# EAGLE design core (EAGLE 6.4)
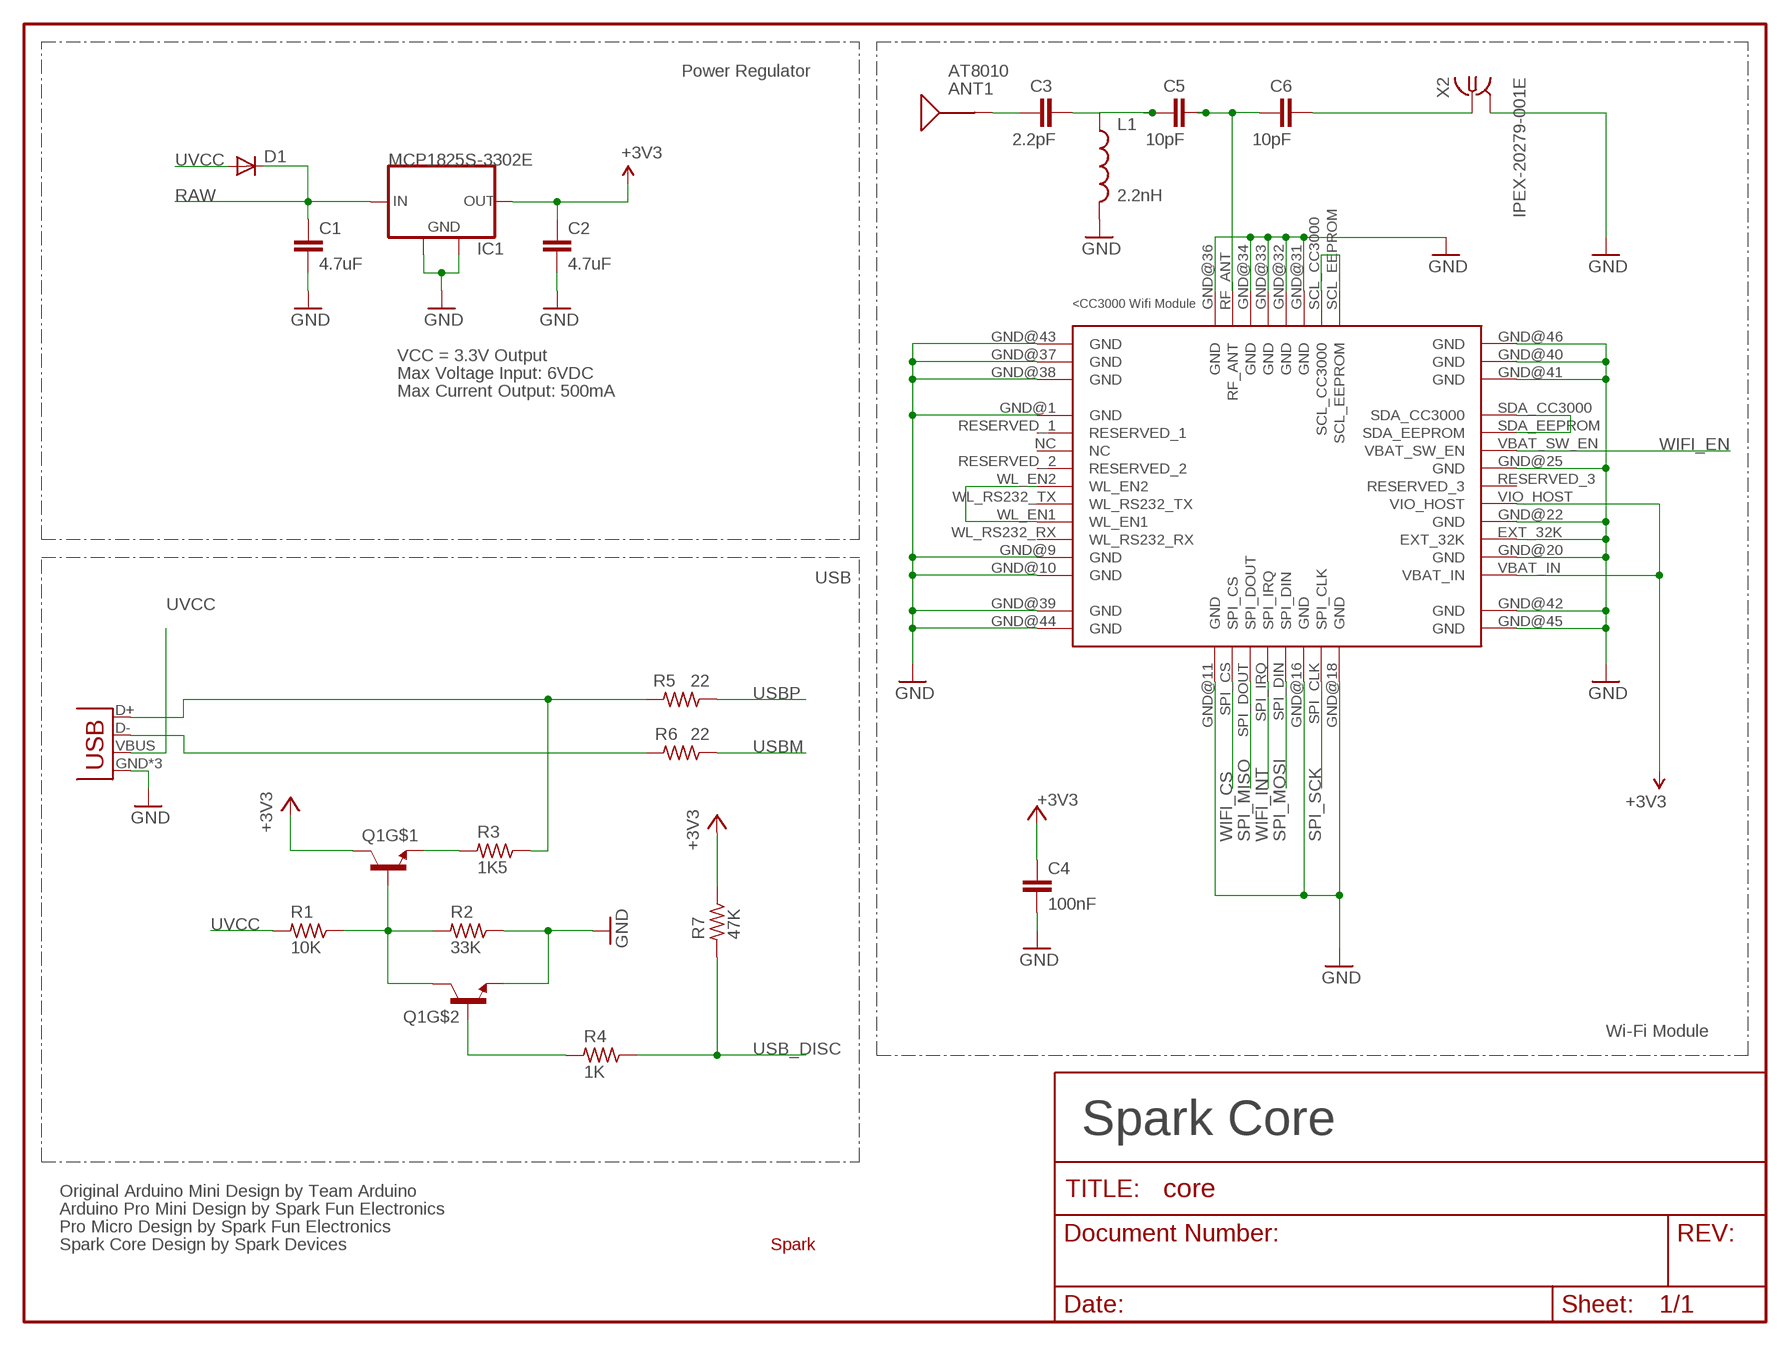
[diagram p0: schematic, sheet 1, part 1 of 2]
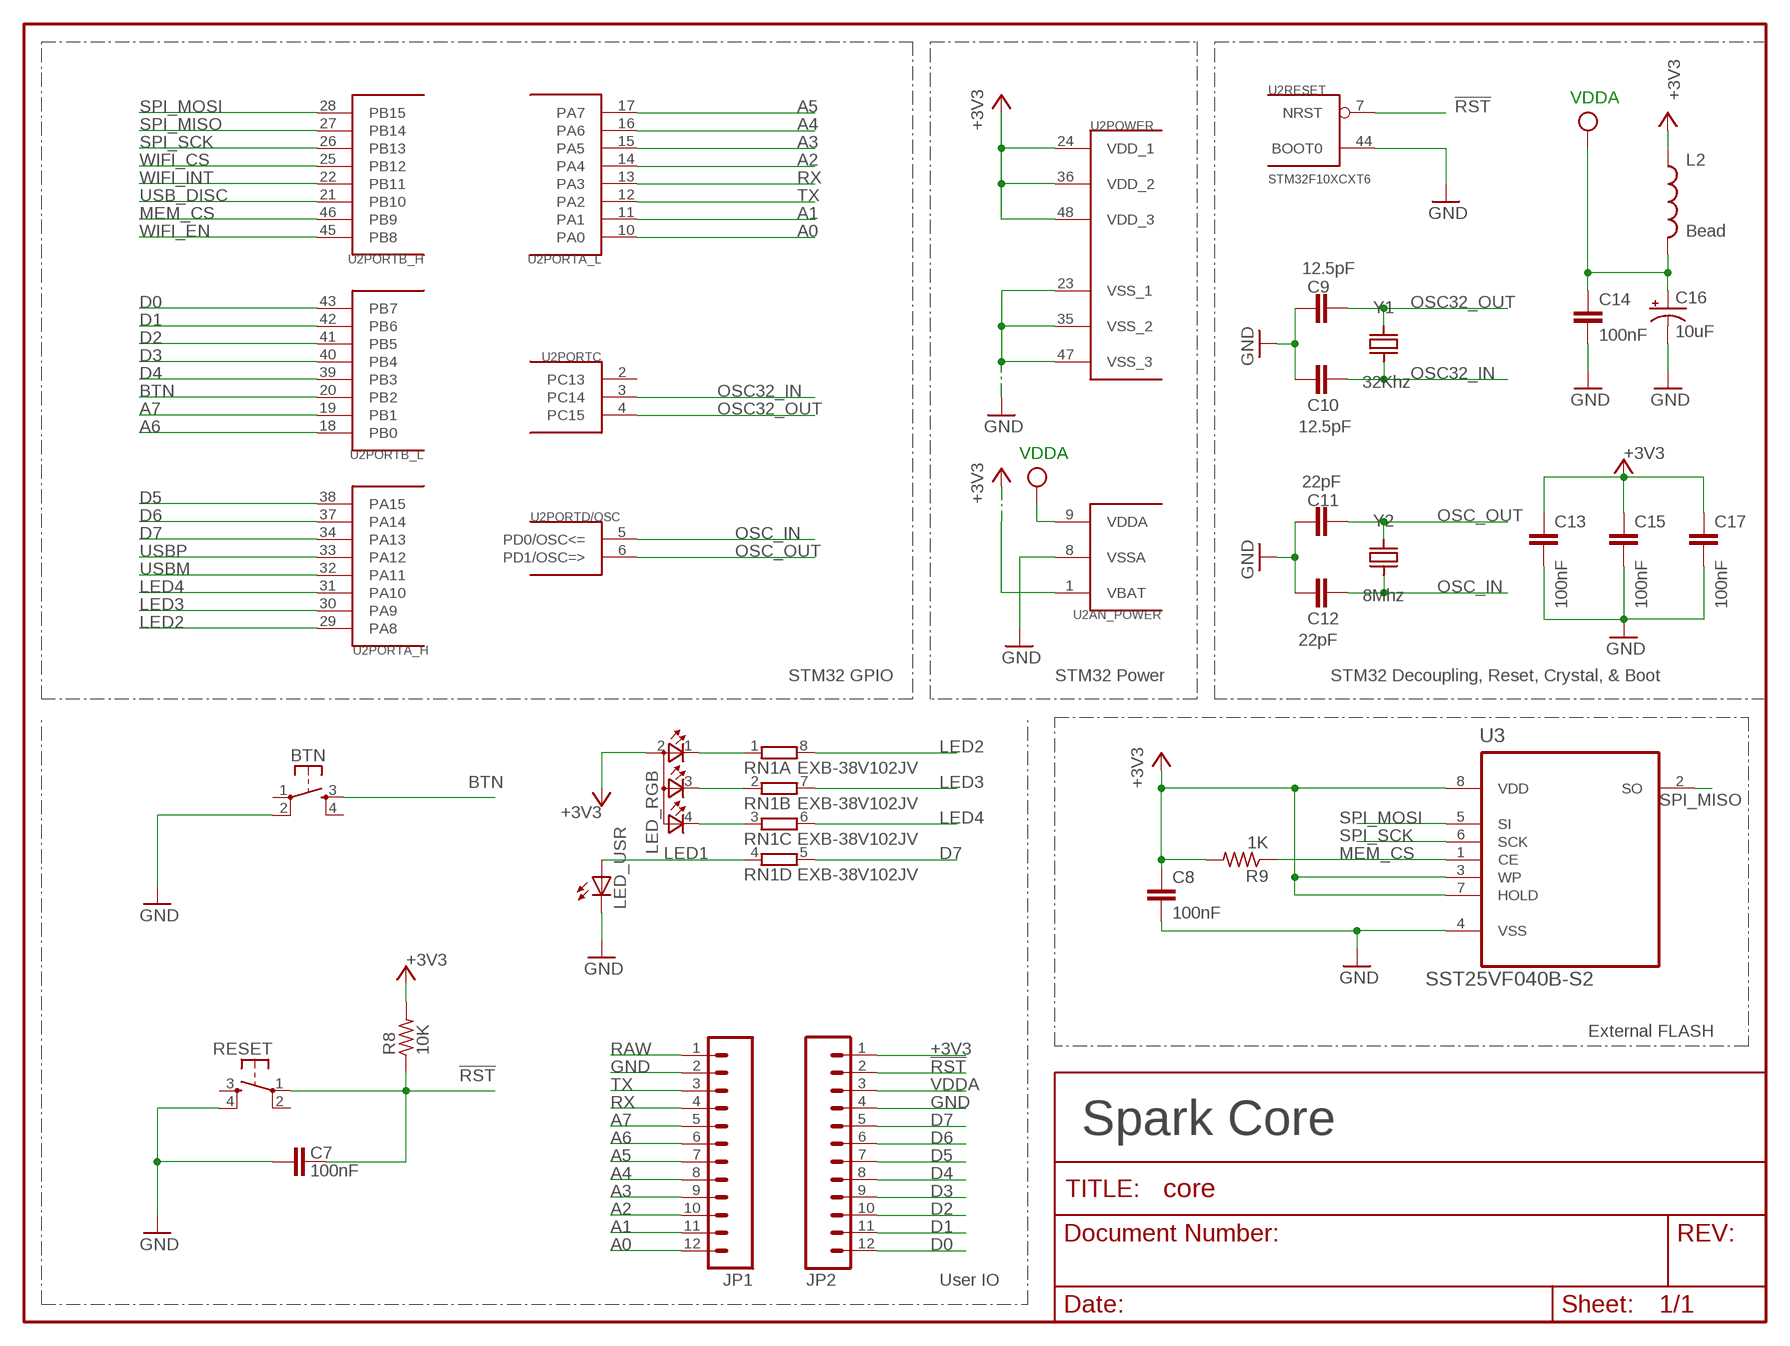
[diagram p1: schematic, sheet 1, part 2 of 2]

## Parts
ANT1  AT8010  [AT8010]
BTN  KMR211GLFS  TAC_SWITCHSMD  [TACTILE_SWITCH_SMD]
C1  4.7uF  C-EUC0603  [C0603]
C2  4.7uF  C-EUC0603  [C0603]
C3  2.2pF  C-EUC0603  [C0603]
C4  100nF  C-EUC0603  [C0603]
C5  10pF  C-EUC0603  [C0603]
C6  10pF  C-EUC0603  [C0603]
C7  100nF  C-EUC0603  [C0603]
C8  100nF  C-EUC0603  [C0603]
C9  12.5pF  C-EUC0603  [C0603]
C10  12.5pF  C-EUC0603  [C0603]
C11  22pF  C-EUC0603  [C0603]
C12  22pF  C-EUC0603  [C0603]
C13  100nF  C-EUC0603  [C0603]
C14  100nF  C-EUC0603  [C0603]
C15  100nF  C-EUC0603  [C0603]
C16  10uF  TANT-CAP1206  [EIA3216]
C17  100nF  C-EUC0603  [C0603]
D1  DIODESOD  [SOD-323]
IC1  MCP1825S-3302E  MCP1825S-SOT223  [SOT223]
JP1  M12PTH  [1X12]
JP2  M12PTH  [1X12]
L1  2.2nH  INDUCTOR0603  [0603]
L2  Bead  INDUCTOR0603  [0603]
LED_RGB  TOPLED-3PLCC  [P-LCC-4-3]
LED_USR  LED0603  [LED-0603]
Q1  MMDT3904  [SOT363]
R1  10K  R-US_R0603  [R0603]
R2  33K  R-US_R0603  [R0603]
R3  1K5  R-US_R0603  [R0603]
R4  1K  R-US_R0603  [R0603]
R5  22  R-US_R0603  [R0603]
R6  22  R-US_R0603  [R0603]
R7  47K  R-US_R0603  [R0603]
R8  10K  R-US_R0603  [R0603]
R9  1K  R-US_R0603  [R0603]
RESET  KMR211GLFS  TAC_SWITCHSMD  [TACTILE_SWITCH_SMD]
RN1  EXB-38V102JV  4R-NEXB38V  [EXB38V]
U1  CC3000  [CC3000]
U2  STM32F10XCXT6  [TQFP48]
U3  SST25VF040B-S2  [SOIC127P790X216-8N]
U$1  SPARK_LOGO2  [SPARK_LOGO2]
X1  USB-MICROB  USBUSB-MICROB-ALIGN  [USB-MICROB-ALIGN]
X2  IPEX-20279-001E  [IPEX-20279-001E]
Y1  32Khz  Q_FC135  [FC135]
Y2  8Mhz  Q_3.2X2.5  [OSC3.2X.2.5]

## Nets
!RST: C7.2 JP2.2 R8.1 RESET.1 U2.7(RESET:NRST)
+3V3: C2.1 C4.1 C8.1 C13.1 C15.1 C17.1 IC1.3(OUT) JP2.1 L2.1 LED_RGB.2(A2) Q1.3(C) R7.1 R8.2 R9.2 U1.VBAT_IN U1.VIO_HOST U2.1(AN_POWER:VBAT) U2.24(POWER:VDD_1) U2.36(POWER:VDD_2) U2.48(POWER:VDD_3) U3.3(WP) U3.7(HOLD) U3.8(VDD)
A0: JP1.12 U2.10(PORTA_L:PA0)
A1: JP1.11 U2.11(PORTA_L:PA1)
A2: JP1.10 U2.14(PORTA_L:PA4)
A3: JP1.9 U2.15(PORTA_L:PA5)
A4: JP1.8 U2.16(PORTA_L:PA6)
A5: JP1.7 U2.17(PORTA_L:PA7)
A6: JP1.6 U2.18(PORTB_L:PB0)
A7: JP1.5 U2.19(PORTB_L:PB1)
BTN: BTN.3 U2.20(PORTB_L:PB2)
D0: JP2.12 U2.43(PORTB_L:PB7)
D1: JP2.11 U2.42(PORTB_L:PB6)
D2: JP2.10 U2.41(PORTB_L:PB5)
D3: JP2.9 U2.40(PORTB_L:PB4)
D4: JP2.8 U2.39(PORTB_L:PB3)
D5: JP2.7 U2.38(PORTA_H:PA15)
D6: JP2.6 U2.37(PORTA_H:PA14)
D7: JP2.5 RN1.5 U2.34(PORTA_H:PA13)
GND [vcc]: BTN.2 C1.2 C2.2 C4.2 C7.1 C8.2 C9.2 C10.2 C11.2 C12.2 C13.2 C14.2 C15.2 C16.C(-) C17.2 IC1.2(GND) IC1.4(GND) JP1.2 JP2.4 L1.2 LED_USR.C Q1.1(E) R2.1 RESET.4 U1.EXT_32K U1.GND@1(GND) U1.GND@9(GND) U1.GND@10(GND) U1.GND@11(GND) U1.GND@16(GND) U1.GND@18(GND) U1.GND@20(GND) U1.GND@22(GND) U1.GND@25(GND) U1.GND@31(GND) U1.GND@32(GND) U1.GND@33(GND) U1.GND@34(GND) U1.GND@36(GND) U1.GND@37(GND) U1.GND@38(GND) U1.GND@39(GND) U1.GND@40(GND) U1.GND@41(GND) U1.GND@42(GND) U1.GND@43(GND) U1.GND@44(GND) U1.GND@45(GND) U1.GND@46(GND) U2.8(AN_POWER:VSSA) U2.23(POWER:VSS_1) U2.35(POWER:VSS_2) U2.44(RESET:BOOT0) U2.47(POWER:VSS_3) U3.4(VSS) X1.GND X1.MT1(GND) X1.MT2(GND) X2.2@1(GND) X2.2@2(GND)
LED1: LED_USR.A RN1.4
LED2: RN1.8 U2.29(PORTA_H:PA8)
LED3: RN1.7 U2.30(PORTA_H:PA9)
LED4: RN1.6 U2.31(PORTA_H:PA10)
MEM_CS: R9.1 U2.46(PORTB_H:PB9) U3.1(CE)
N$1: R3.1 R5.2 X1.D+
N$2 [RF]: C6.2 X2.1
N$3 [RF]: ANT1.SIG(SIGNAL) C3.1
N$4 [RF]: C5.2 C6.1 U1.RF_ANT
N$5 [RF]: C3.2 C5.1 L1.1
N$6: R6.2 X1.D-
N$7: U1.SCL_CC3000 U1.SCL_EEPROM
N$8: Q1.2(B) R4.2
N$9: U1.WL_EN1 U1.WL_EN2
N$10: LED_RGB.1(CRED) RN1.1
N$12: LED_RGB.3(CBLUE) RN1.2
N$13: Q1.5(B) Q1.6(C) R1.1 R2.2
N$14: LED_RGB.4(CGREEN) RN1.3
N$15: U1.SDA_CC3000 U1.SDA_EEPROM
N$16: Q1.4(E) R3.2
OSC32_IN: C10.1 U2.3(PORTC:PC14) Y1.X1
OSC32_OUT: C9.1 U2.4(PORTC:PC15) Y1.X2
OSC_IN: C12.1 U2.5(PORTD/OSC:PD0/OSC<=) Y2.P$1
OSC_OUT: C11.1 U2.6(PORTD/OSC:PD1/OSC=>) Y2.P$3
RAW [vcc]: C1.1 D1.1(C) IC1.1(IN) JP1.1
RX: JP1.4 U2.13(PORTA_L:PA3)
SPI_MISO: U1.SPI_DOUT U2.27(PORTB_H:PB14) U3.2(SO)
SPI_MOSI: U1.SPI_DIN U2.28(PORTB_H:PB15) U3.5(SI)
SPI_SCK: U1.SPI_CLK U2.26(PORTB_H:PB13) U3.6(SCK)
TX: JP1.3 U2.12(PORTA_L:PA2)
USB_DISC: R4.1 R7.2 U2.21(PORTB_H:PB10)
USBM: R6.1 U2.32(PORTA_H:PA11)
USBP: R5.1 U2.33(PORTA_H:PA12)
UVCC: D1.2(A) R1.2 X1.VBUS
VDDA: C14.1 C16.A(+) JP2.3 L2.2 U2.9(AN_POWER:VDDA) ; supply symbol labelled VCC
WIFI_CS: U1.SPI_CS U2.25(PORTB_H:PB12)
WIFI_EN: U1.VBAT_SW_EN U2.45(PORTB_H:PB8)
WIFI_INT: U1.SPI_IRQ U2.22(PORTB_H:PB11)
Unconnected: BTN.1 BTN.4 RESET.2 RESET.3 U1.NC U1.RESERVED_1 U1.RESERVED_2 U1.RESERVED_3 U1.WL_RS232_RX U1.WL_RS232_TX U2.2(PORTC:PC13)

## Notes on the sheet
- Power Regulator
- VDDA
- VCC = 3.3V Output
- Max Voltage Input: 6VDC
- Max Current Output: 500mA
- VDDA
- USB
- STM32 GPIO | STM32 Power | STM32 Decoupling, Reset, Crystal, & Boot
- Wi-Fi Module | External FLASH
- Spark Core | Spark Core
- Original Arduino Mini Design by Team Arduino
- Arduino Pro Mini Design by Spark Fun Electronics
- Pro Micro Design by Spark Fun Electronics
- Spark Core Design by Spark Devices
- User IO

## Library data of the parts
ANT1 = Spark:AT8010: AT8010 Series Multilayer Chip Antenna
BTN RESET = Spark:TAC_SWITCH: SMD Tactiile Switch
C1-C15 C17 = rcl:C-EU: CAPACITOR, European symbol
C16 = Spark:TANT-CAP: Tantalum SMT
D1 = SparkFun:DIODE: Diode
IC1 = Spark:MCP1825S: 500 mA, Low Voltage, Low Quiescent Current LDO Regulator
JP1 JP2 = SparkFun:M12: Header 12 Standard 12-pin 0.1" header. Use with straight break away headers (SKU : PRT-00116), right angle break away headers (PRT-00553), swiss pins (PRT-00743), machine pins (PRT-00117), and female headers (PRT-00115).
L1 L2 = SparkFun-Passives:INDUCTOR: Inductors
LED_RGB = Spark:TOPLED-3: Cree CLVBA-FKA
LED_USR = SparkFun:LED: LEDs
Q1 = SparkFun-DiscreteSemi:MMDT3904: Dual NPN transistor
R1-R9 = rcl:R-US_: RESISTOR, American symbol
RN1 = resistor-dil:4R-N: Array Chip Resistor Source: RS Component / Phycomp; OC_FARNELL: unknown; OC_NEWARK: unknown
U1 = CC3000:CC3000
U2 = stm32:STM32F10XCXT6: ST STM32F101/103 48pin LQFP
U3 = Spark:SST25VF040B: 4 Mbit SPI Serial Flash
U$1 = Spark:SPARK_LOGO2
X1 = Spark:USB: USB Connectors USB-B-PTH is fully proven SKU : PRT-00139/CONN-08278 USB-miniB is fully proven SKU : PRT-00587 USB-A-PCB is untested. USB-A-H is throughly reviewed, but untested. Spark Fun Electronics SKU : PRT-00437 USB-B-SMT is throughly reviewed, but untested. Needs silkscreen touching up.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
X2 = Spark:IPEX-20279-001E: Ultra Miniature Coaxial SMT RF Receptacle
Y1 Y2 = Spark:Q

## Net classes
2 RF: width 0.635 mm, clearance 0.762 mm

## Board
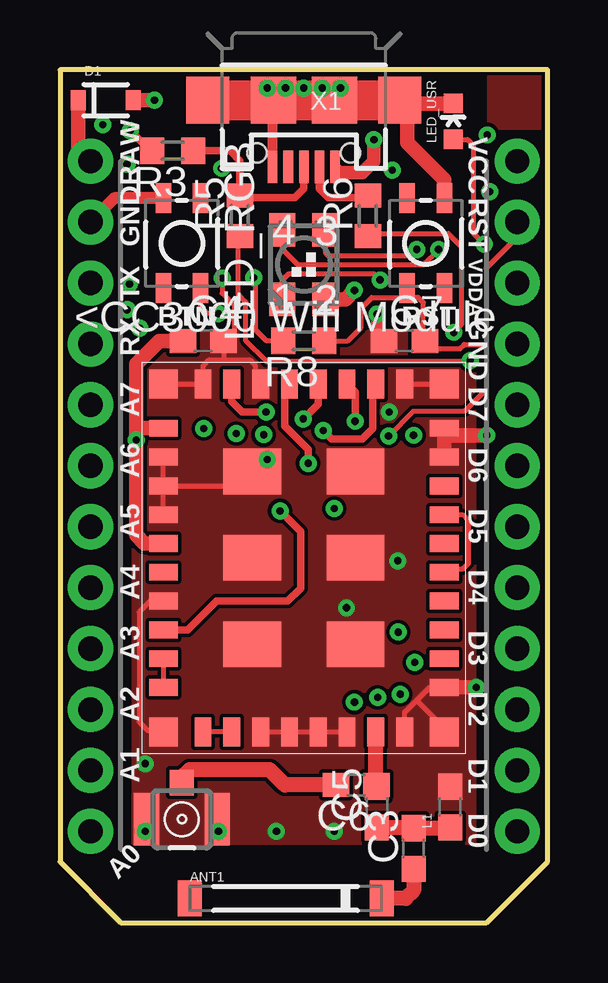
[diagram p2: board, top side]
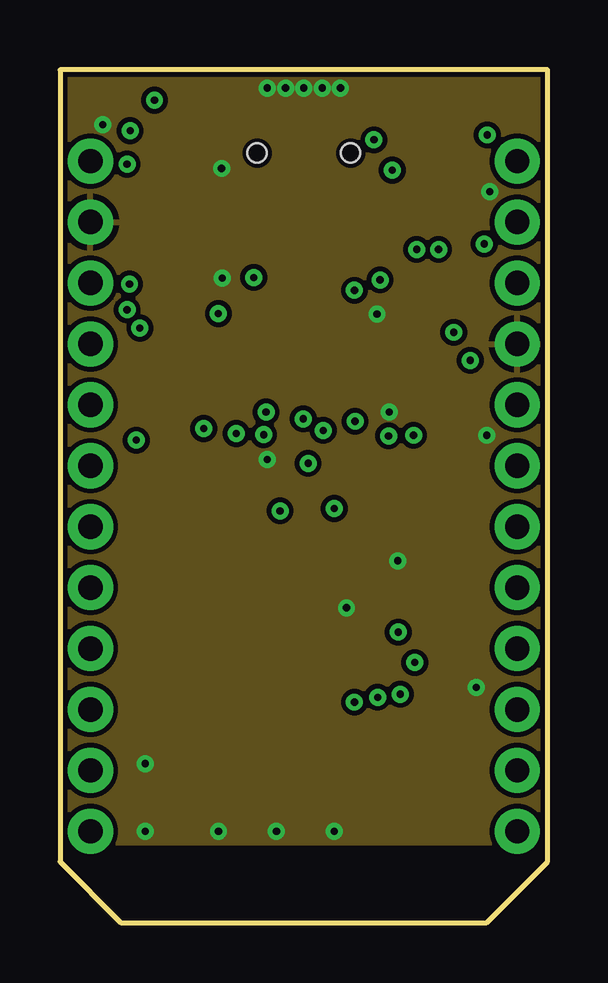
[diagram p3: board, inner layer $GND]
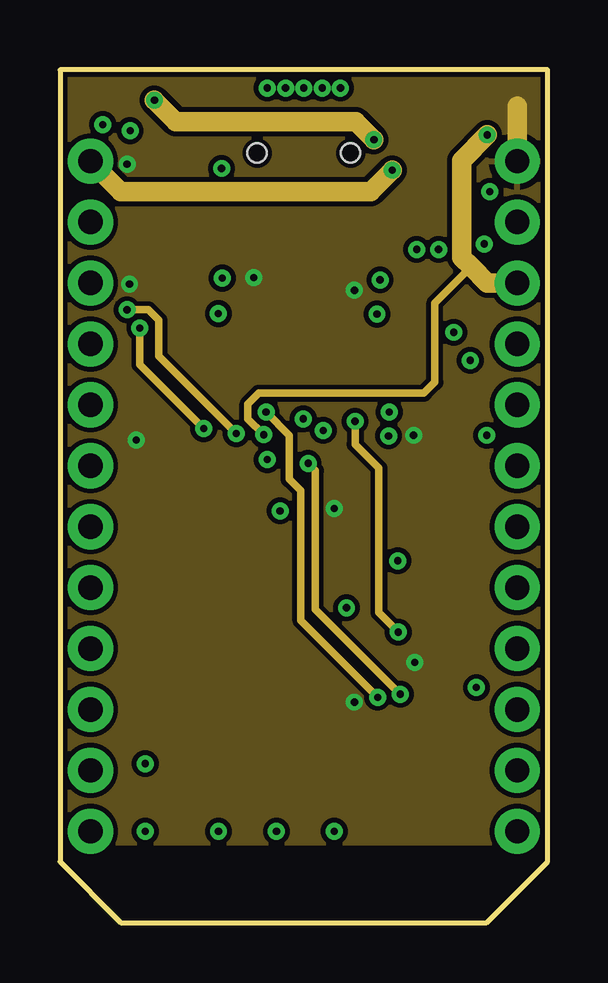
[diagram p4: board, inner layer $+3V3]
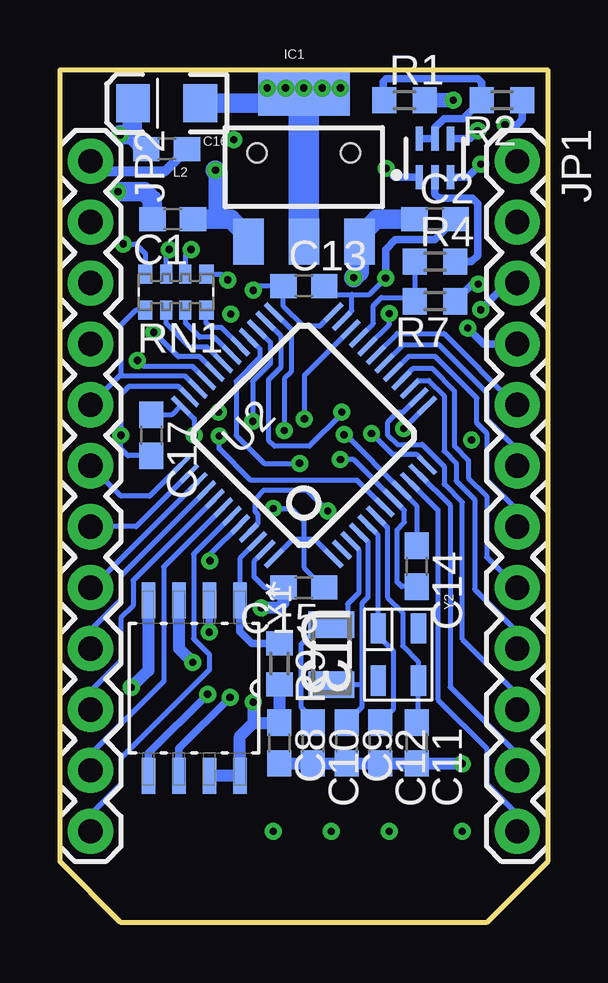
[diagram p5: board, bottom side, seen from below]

Size 20.32 x 35.56 mm. Coordinates in mm from the lower left corner, seen from the top.
Outline: 0,35.56 0,2.54 2.54,0 17.78,0 20.32,2.54 20.32,35.56 0,35.56
Copper layers (1+2*15+16): Top 0.035mm / dielectric 1.5mm / $GND 0.035mm / dielectric 0.15mm / $+3V3 0.035mm / dielectric 0.2mm / Bottom 0.035mm
Design rules "spark": minimum track width 6mil, minimum drill 0.3mm, track to track 6mil, track to pad 6mil, pad to pad 6mil, via to via 6mil, smd to smd 6mil, copper to edge 6mil, drill to drill 6mil, minimum pad ring 12mil, minimum via ring 8mil, stop-mask expansion 4mil, vias tented up to drill 20mil, thermal gap 10mil

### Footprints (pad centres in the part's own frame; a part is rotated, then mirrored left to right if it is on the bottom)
AT8010 = smd 1 x 1.5: NC -4,0; SIG 4,0
TACTILE_SWITCH_SMD = smd 1.25 x 0.65: 1 -1.875,0.775; 2 1.875,0.775; 3 -1.875,-0.775; 4 1.875,-0.775
C0603 = smd 1.1 x 1: 1 -0.85,0; 2 0.85,0
EIA3216 = smd 1.4 x 1.6: A 1.4,0; C -1.4,0
SOD-323 = smd 0.63 x 0.83: 1 -1.15,0; 2 1.15,0
SOT223 = smd 1.27 x 1.905: 1 -2.311,-3.099; 2 0,-3.099; 3 2.311,-3.099 | smd 3.81 x 1.905: 4 0,3.099
1X12 = drill 1.016 pad 1.88: 1 0,0; 2 2.54,0; 3 5.08,0; 4 7.62,0; 5 10.16,0; 6 12.7,0; 7 15.24,0; 8 17.78,0; 9 20.32,0; 10 22.86,0; 11 25.4,0; 12 27.94,0
0603 = smd 1.1 x 1: 1 -0.85,0; 2 0.85,0
P-LCC-4-3 = smd 1.1 x 1.4: 1 -0.9,-1.45; 2 0.9,-1.45; 3 0.9,1.45; 4 -0.9,1.45
LED-0603 = smd 0.8 x 0.8: A 0,-0.75; C 0,0.75
SOT363 = smd 0.3 x 0.99: 1 -0.65,-0.8; 2 0,-0.8; 3 0.65,-0.8; 4 0.65,0.81; 5 0,0.81; 6 -0.65,0.81
R0603 = smd 1 x 1.1: 1 -0.85,0; 2 0.85,0
EXB38V = smd 0.6 x 0.8: 1 -1.275,-0.75; 4 1.275,-0.75; 5 1.275,0.75; 8 -1.275,0.75 | smd 0.5 x 0.8: 2 -0.4,-0.75; 3 0.4,-0.75; 6 0.4,0.75; 7 -0.4,0.75
CC3000 = smd 1.2 x 0.7: EXT_32K 5.85,-2.97; GND@1 -5.85,5.43; GND@9 -5.85,-4.17; GND@10 -5.85,-5.37; GND@20 5.85,-4.17; GND@22 5.85,-1.77; GND@25 5.85,1.83; NC -5.85,3.03; RESERVED_1 -5.85,4.23; RESERVED_2 -5.85,1.83; RESERVED_3 5.85,0.63; SDA_CC3000 5.85,5.43; SDA_EEPROM 5.85,4.23; VBAT_IN 5.85,-5.37; VBAT_SW_EN 5.85,3.03; VIO_HOST 5.85,-0.57; WL_EN1 -5.85,-1.77; WL_EN2 -5.85,0.63; WL_RS232_RX -5.85,-2.97; WL_RS232_TX -5.85,-0.57 | smd 0.7 x 1.2: GND@11 -4.2,-7.22; GND@16 1.8,-7.22; GND@18 4.2,-7.22; GND@31 1.8,7.28; GND@32 0.6,7.28; GND@33 -0.6,7.28; GND@34 -1.8,7.28; GND@36 -4.2,7.28; RF_ANT -3,7.28; SCL_CC3000 3,7.28; SCL_EEPROM 4.2,7.28; SPI_CLK 3,-7.22; SPI_CS -3,-7.22; SPI_DIN 0.6,-7.22; SPI_DOUT -1.8,-7.22; SPI_IRQ -0.6,-7.22 | smd 2.4 x 1.9: GND@37 -2.15,3.63; GND@38 -2.15,0.03; GND@39 -2.15,-3.57; GND@40 2.15,3.63; GND@41 2.15,0.03; GND@42 2.15,-3.57 | smd 1.2 x 1.2: GND@43 -5.85,7.28; GND@44 -5.85,-7.22; GND@45 5.85,-7.22; GND@46 5.85,7.28
TQFP48 = smd 0.2 x 1: 1 -2.75,-4.5; 2 -2.25,-4.5; 3 -1.75,-4.5; 4 -1.25,-4.5; 5 -0.75,-4.5; 6 -0.25,-4.5; 7 0.25,-4.5; 8 0.75,-4.5; 9 1.25,-4.5; 10 1.75,-4.5; 11 2.25,-4.5; 12 2.75,-4.5; 25 2.75,4.5; 26 2.25,4.5; 27 1.75,4.5; 28 1.25,4.5; 29 0.75,4.5; 30 0.25,4.5; 31 -0.25,4.5; 32 -0.75,4.5; 33 -1.25,4.5; 34 -1.75,4.5; 35 -2.25,4.5; 36 -2.75,4.5 | smd 1 x 0.2: 13 4.5,-2.75; 14 4.5,-2.25; 15 4.5,-1.75; 16 4.5,-1.25; 17 4.5,-0.75; 18 4.5,-0.25; 19 4.5,0.25; 20 4.5,0.75; 21 4.5,1.25; 22 4.5,1.75; 23 4.5,2.25; 24 4.5,2.75; 37 -4.5,2.75; 38 -4.5,2.25; 39 -4.5,1.75; 40 -4.5,1.25; 41 -4.5,0.75; 42 -4.5,0.25; 43 -4.5,-0.25; 44 -4.5,-0.75; 45 -4.5,-1.25; 46 -4.5,-1.75; 47 -4.5,-2.25; 48 -4.5,-2.75
SOIC127P790X216-8N = smd 1.499 x 0.559: 1 -3.658,1.905; 2 -3.658,0.635; 3 -3.658,-0.635; 4 -3.658,-1.905; 5 3.658,-1.905; 6 3.658,-0.635; 7 3.658,0.635; 8 3.658,1.905
USB-MICROB-ALIGN = smd 0.4 x 1.35: D+ 0,2.775; D- -0.65,2.775; GND 1.3,2.775; ID 0.65,2.775; VBUS -1.3,2.775 | smd 1.8 x 1.95: MT1 -4,0; MT2 4,0 | smd 1.9 x 1.95: P$1 -1.27,0; P$2 1.27,0 | hole 0.8: -1.95,2.2; 1.95,2.2
IPEX-20279-001E = smd 1 x 1.05: 1 0,1.528 | smd 1.05 x 2.2: 2@1 -1.475,0; 2@2 1.475,0
FC135 = smd 1.1 x 1.9: X1 -1.25,0; X2 1.25,0
OSC3.2X.2.5 = smd 1.27 x 0.635: P$1 -1.092,-0.838; P$2 1.092,-0.838; P$3 1.092,0.838; P$4 -1.092,0.838

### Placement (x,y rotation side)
ANT1  9.4,1.02 0 top
BTN  5.08,28.32 90 top
C1  15.62,29.34 180 bottom
C2  4.7,29.34 0 bottom
C3  14.73,3.1 90 top
C4  5.97,24.26 0 top
C5  13.21,4.83 90 top
C6  12.34,5.74 180 top
C7  14.35,24.26 0 top
C8  11.18,7.49 270 bottom
C9  8.38,7.49 270 bottom
C10  9.78,7.49 270 bottom
C11  5.46,7.49 270 bottom
C12  6.99,7.49 270 bottom
C13  10.16,26.54 0 bottom
C14  5.46,14.86 270 bottom
C15  10.16,13.97 180 bottom
C16  15.88,34.16 180 bottom
C17  16.51,20.32 270 bottom
D1  1.91,34.29 0 top
IC1  10.16,31.5 0 bottom
JP1  1.27,31.75 270 bottom
JP2  19.05,31.75 270 bottom
L1  16.26,4.83 90 top
L2  15.88,32.26 180 bottom
LED_RGB  10.16,27.43 0 top
LED_USR  16.38,33.4 0 top
Q1  4.7,31.88 0 bottom
R1  5.97,34.29 0 bottom
R2  1.91,34.29 180 bottom
R3  4.7,32.18 180 top
R4  4.7,27.56 0 bottom
R5  7.49,29.46 90 top
R6  12.83,29.46 90 top
R7  4.7,25.91 180 bottom
R8  10.16,24.26 180 top
R9  11.18,10.8 270 bottom
RESET  15.24,28.32 90 top
RN1  15.49,26.29 180 bottom
U1  10.16,15.24 180 top
U2  10.16,20.32 45 bottom
U3  14.73,9.78 270 bottom
U$1  17.78,33.02 0 top
X1  10.16,34.29 180 top
X2  5.08,4.32 0 top
Y1  9.02,11.18 270 bottom
Y2  6.22,11.18 270 bottom

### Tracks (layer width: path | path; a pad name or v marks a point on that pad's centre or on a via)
!RST  (via drill 0.3)
  Top 0.203: 17.75,24.08 17.75,27.28 19.05,28.57 JP2.2 | 17.75,24.08 17.75,22.22 16.84,21.31 14.71,21.31 v13.69,20.29 | 17.75,24.08 17.73,24.11 16.84,24.11 16.66,23.93 15.53,23.93 C7.2 15.14,24.32 15.14,25.86 14.94,26.06 14.46,26.06 | R8.1 11.99,24.26 12.55,24.82 12.55,25.63 12.98,26.06 14.46,26.06 | 14.46,26.06 RESET.1
  Bottom 0.203: U2.7 7.93,18.44 12.37,18.44 13.69,19.76 v13.69,20.29
+3V3  (via drill 0.3)
  Top 0.203: R8.2 8.61,24.26 8.15,24.71 8.15,26.82 v8.08,26.9
  Top 0.61: U1.VIO_HOST 3.52,15.81 3.17,16.15 v3.17,20.12 3.17,20.62 | 3.17,20.62 3.17,23.29 4.14,24.26 C4.1 | U1.VBAT_IN 4.29,20.62 3.17,20.62 | LED_RGB.2 11.88,25.98 v12.27,26.36
  $+3V3 0.813: JP2.1 19.05,34.04
  Bottom 0.203: U2.1 9.71,15.98 10.16,15.98 | 10.16,15.98 10.62,15.98 U2.48 | v11.43,17.27 10.69,17.27 10.16,16.74 10.16,15.98 | 9.32,13.97 C15.1 10.16,14.82 10.16,15.98 | v12.27,26.36 12.09,26.54 C13.1 11.01,25.69 10.19,24.87 9.5,24.87 U2.24 | C17.1 15.67,21.17 U2.36 14.73,21 v14.73,20.32
  Bottom 0.305: R7.1 3.14,26.62 v2.9,26.62 | Q1.3 3.34,31.08 v2.79,31.62
  Bottom 0.406: L2.1 15.96,31.32 18.62,31.32 JP2.1
  Bottom 0.508: 12.27,8.33 12.83,7.77 U3.8 U3.7 | 12.27,8.33 C8.1 R9.2 | v12.27,9.2 12.27,8.33 | U3.3 15.37,11.43 v14.78,10.85
  Bottom 0.813: C2.1 7.11,29.34 7.85,28.6 IC1.3 7.85,27.13 v8.08,26.9
  pour $+3V3 (isolate 0.203): 0,35.56 20.32,35.56 20.32,3.3 0,3.3
A0
  Bottom 0.203: U2.10 4.57,17.21 4.57,9.3 2.54,7.26 2.54,5.79 1.27,4.52 JP1.12
A1
  Bottom 0.203: U2.11 4.06,17.41 4.06,9.83 1.27,7.04 JP1.11
A2
  Bottom 0.203: U2.14 6.04,21.26 6.27,21.26 6.66,20.88 6.66,20.32 6.27,19.94 5.23,19.94 4.32,19.02 4.32,18.29 3.56,17.53 3.56,11.81 1.27,9.53 JP1.10
A3
  Bottom 0.203: U2.15 5.4,22.61 4.95,22.61 4.32,21.97 4.32,19.66 3.81,19.15 3.81,18.41 3.05,17.65 3.05,13.89 1.27,12.12 JP1.9
A4
  Bottom 0.203: U2.16 5.6,23.11 4.83,23.11 3.89,22.17 3.89,19.86 3.3,19.28 3.3,18.54 2.54,17.78 2.54,15.24 JP1.8
A5
  Bottom 0.203: U2.17 5.8,23.62 4.7,23.62 2.95,21.87 2.95,20.83 2.54,20.42 2.54,18.47 1.27,17.2 JP1.7
A6
  Bottom 0.203: U2.18 6.02,24.11 4.55,24.11 2.54,22.1 2.54,21.01 1.27,19.74 JP1.6
A7
  Bottom 0.203: U2.19 6.27,24.56 4.32,24.56 1.35,21.59 JP1.5
BTN  (via drill 0.3)
  Top 0.203: 5.84,26.43 BTN.3 5.87,26.43 5.87,25.65 6.13,25.39 v6.6,25.39
  Bottom 0.203: U2.20 6.6,24.94 v6.6,25.39
D0
  Bottom 0.203: U2.43 14.76,15.37 14.76,11.84 14.1,11.18 14.1,10.54 17.78,6.86 17.78,5.77 19.05,4.5 JP2.12
D1
  Bottom 0.203: U2.42 16,14.83 16,10.06 19.05,7.01 JP2.11
D2
  Bottom 0.203: JP2.10 19.05,9.65 17.78,10.92 17.78,12.7 17.27,13.21 17.27,14.27 U2.41
D3
  Bottom 0.203: JP2.9 19.05,12.19 17.78,13.46 17.78,14.48 17.77,14.48 U2.40
D4
  Bottom 0.203: U2.39 18.98,13.97 JP2.8
D5
  Bottom 0.203: JP2.7 17.15,16.51 U2.38
D6
  Bottom 0.203: U2.37 16.59,17.78 17.78,17.78 JP2.6
D7
  Bottom 0.203: U2.34 15.1,22.78 17.86,22.78 | 17.86,22.78 JP2.5 | RN1.5 17.16,25.54 17.78,24.92 17.78,22.86 17.86,22.78
GND  (via drill 0.3)
  Top 0.203: U1.GND@43 16.01,8.12 14.86,9.27 | U1.GND@36 14.36,8.77 14.86,9.27 | U1.GND@1 15.4,9.81 14.86,9.27 | v8.64,19.3 8.14,18.81 U1.GND@42 7.41,18.21 U1.EXT_32K | U1.GND@34 U1.GND@33 U1.GND@32 U1.GND@31 8.36,8.4 | U1.GND@22 U1.EXT_32K | U1.GND@45 U1.GND@18 | U1.GND@38 12.41,15.11 | U1.GND@25 4.49,13.59 3.94,13.59 3.3,12.95 3.3,8.38 3.68,8 4.27,8 U1.GND@46 | U1.GND@11 U1.GND@44 | U1.EXT_32K U1.GND@20 | U1.GND@18 | 8.26,21.97 8.26,22.36 U1.GND@16 8.13,22.69 8.13,23.24 7.9,23.47 6.83,23.47 | 6.22,34.23 X1.MT2 | U1.GND@18 5.96,23.21 6.22,23.47 6.83,23.47 | 6.83,23.47 6.82,23.48 C4.2 7.26,24.7 7.26,25.73 6.76,26.24 v6.76,26.87
  Top 0.305: 14.16,34.15 X1.MT1
  Top 0.406: X1.GND 8.86,34.26 8.89,34.29 8.89,34.54 v8.64,34.8
  Top 0.508: v13.21,25.38 13.21,24.55 C7.1 | BTN.2 2.26,30.2 JP1.2
  Top 0.61: U1.GND@1 v17.34,9.81 v17.35,9.8 | U1.GND@9 U1.GND@10 16.3,20.32 v17.78,20.32 | LED_USR.C 14.3,34.15 X1.MT1 14.48,33.97 14.48,32.51 16.02,30.97 RESET.4
  Top 0.813: 6.22,34.23 6.29,34.29
  Top 1.676: 6.29,34.29 8.89,34.29 X1.MT1
  Bottom 0.203: U2.35 15.37,22.35 17.45,22.35 17.78,22.02 v17.78,20.32 17.78,19.76 17.49,19.47 C17.2 | v8.64,19.3 8.08,19.3 U2.8 5.97,17.19 5.97,16.69 6.27,16.38 6.27,14.2 6.08,14.01 C14.2 | U2.44 14.07,15.35 v14.07,15.09 | U2.47 12.24,15.05 12.24,14.43 11.79,13.97 C15.2 | C13.2 8.95,26.19 8.15,26.19 | 8.15,26.19 7.44,26.19 v6.76,26.87 | U2.23 8.15,25.51 8.15,26.19
  Bottom 0.305: 10.16,34.67 IC1.4 | 1.02,34.29 R2.1 1.05,33.49 1.27,33.27 v1.78,33.27 | Q1.1 6.36,31.08 v6.73,31.45 | C2.2 4.71,28.47 6.35,28.47 6.76,28.07 v6.76,26.87
  Bottom 0.508: U3.4 16.64,10.52 v17.35,9.8 | v3.56,6.63 3.57,6.64 C11.2 C12.2 C9.2 C10.2 C8.2 | C15.2 11.01,13.32 11.2,13.13 v11.94,13.13
  Bottom 0.813: 10.46,34.29 IC1.4 | C1.2 16.47,30.14 16.82,30.48 v17.91,30.48 | v10.16,34.8 IC1.4 | C16.C 10.59,34.16 IC1.4
  Bottom 1.27: IC1.2 IC1.4
  other vias: 3.56,3.81 6.6,3.81 9.02,3.81 11.43,3.81 13.72,21.29 11.68,34.8 10.92,34.8 9.4,34.8
  pour $GND (isolate 0.203): 0,35.56 20.32,35.56 20.32,3.3 0,3.3
  pour Top (no thermals): 3.05,3.3 3.05,24.64 17.27,24.64 17.27,3.3
LED1  (via drill 0.3)
  Top 0.203: LED_USR.A 16.98,32.65 17.22,32.41 17.22,28.75 v17.68,28.3
  Bottom 0.203: v17.68,28.3 17.17,28.3 16.76,27.89 RN1.4
LED2
  Bottom 0.203: U2.29 13.6,24.82 14.05,24.82 14.22,24.99 RN1.8
LED3
  Bottom 0.203: U2.30 13.9,24.41 14.5,24.41 15.09,24.99 RN1.7
LED4
  Bottom 0.203: U2.31 14.2,24 14.91,24 15.9,24.99 RN1.6
MEM_CS
  Bottom 0.203: U2.46 12.83,15.18 U3.1
  Bottom 0.305: R9.1 12.33,11.64 12.83,12.14 U3.1
N$1
  Top 0.305: X1.D+ 10.16,30.61 9.78,30.23 7.58,30.23 R5.2 7.49,31.77 7.09,32.18 R3.1
N$2
  Top 0.635: C6.2 9.37,5.74 8.74,6.38 5.4,6.38 5.08,6.06 X2.1
N$3
  Top 0.635: C3.1 14.73,1.33 14.41,1.02 ANT1.SIG
N$4
  Top 0.406: 13.21,5.74 C6.1
  Top 0.635: C6.1 13.16,5.78 U1.RF_ANT | 13.21,5.74 C5.2
N$5
  Top 0.635: C5.1 14.71,3.98 C3.2 16.23,3.95 L1.1
N$6
  Top 0.305: X1.D- 10.81,30.59 11.18,30.23 12.74,30.23 R6.2
N$7
  Top 0.203: U1.SCL_CC3000 U1.SCL_EEPROM
N$8
  Bottom 0.305: Q1.2 4.7,30.38 4.52,30.2 3.15,30.2 2.92,29.97 2.92,27.81 3.17,27.56 R4.2
N$9
  Top 0.203: U1.WL_EN1 16.77,17.01 17.02,16.76 17.02,14.99 16.76,14.73 16.13,14.73 U1.WL_EN2
N$10  (via drill 0.3)
  Top 0.203: LED_RGB.1 9.26,26.79 9.53,27.05 13.08,27.05 v13.34,26.8
  Bottom 0.203: RN1.1 13.58,27.04 v13.34,26.8
N$11
  pour Top: 17.91,35.56 20.32,35.56 20.32,33.15 17.91,33.15
N$12  (via drill 0.3)
  Top 0.203: LED_RGB.3 11.06,27.93 11.18,27.81 14.61,27.81 v14.86,28.07
  Bottom 0.203: v14.86,28.07 15.09,27.83 RN1.2
N$13
  Bottom 0.305: R1.1 6.86,34.33 6.86,35.05 6.73,35.18 2.92,35.18 2.75,35.01 R2.2 3.52,33.53 4.32,33.53 4.7,33.15 Q1.5 Q1.6
N$14  (via drill 0.3)
  Top 0.203: LED_RGB.4 9.26,28.08 9.91,27.43 15.14,27.43 v15.77,28.07
  Bottom 0.203: RN1.3 15.89,27.95 v15.77,28.07
N$15
  Top 0.203: U1.SDA_EEPROM U1.SDA_CC3000
N$16  (via drill 0.3)
  Top 0.305: R3.2 3.76,32.18 v2.92,33.02
  Bottom 0.305: Q1.4 3.25,32.69 v2.92,33.02
OSC32_IN
  Bottom 0.203: C10.1 10.11,8.67 10.11,8.81 10.29,8.99 10.29,11.58 9.68,12.19 9.25,12.19 Y1.X1 8.82,12.62 8.41,12.62 8.33,12.7 8.33,13.28 7.87,13.74 7.87,15.56 U2.3
OSC32_OUT
  Bottom 0.203: 7.75,9.93 7.75,13.31 7.49,13.56 7.49,15.89 U2.4 | 7.75,9.93 7.75,8.98 C9.1 | Y1.X2 7.75,9.93
OSC_IN
  Bottom 0.203: 7.04,12.29 Y2.P$1 | Y2.P$1 7.06,11.96 6.43,11.33 6.43,8.9 C12.1 | U2.5 7.09,16.19 7.09,12.29 Y2.P$1
OSC_OUT
  Bottom 0.203: C11.1 5.38,8.42 Y2.P$3 5.38,10.87 6.04,11.53 6.04,12.93 6.68,13.56 6.68,16.49 U2.6
RAW  (via drill 0.3)
  Top 0.61: D1.1 0.76,32.27 JP1.1
  $+3V3 0.813: JP1.1 2.54,30.48 12.95,30.48 v13.84,31.37
  Bottom 0.813: IC1.1 12.47,28.6 13.21,29.34 13.72,29.34 | 13.72,29.34 C1.1 | v13.84,31.37 13.72,31.24 13.72,29.34
RX  (via drill 0.3)
  $+3V3 0.305: v3.33,24.79 3.33,23.26 v5.99,20.6
  Bottom 0.203: U2.13 v5.99,20.6
  Bottom 0.305: JP1.4 2.67,24.13 v3.33,24.79
SPI_MISO  (via drill 0.3)
  Top 0.305: U1.SPI_DOUT 12.29,22.13 v12.29,20.9
  $+3V3 0.305: v14.1,12.12 13.28,12.93 13.28,18.95 12.29,19.94 v12.29,20.9
  Bottom 0.203: U2.27 11.56,24.19 11.56,23.32 12.29,22.58 v12.29,20.9
  Bottom 0.305: U3.2 v14.1,12.12
SPI_MOSI  (via drill 0.3)
  Top 0.305: v10.34,19.15 10.34,19.74 9.37,20.7 9.37,22.27 U1.SPI_DIN
  $+3V3 0.305: v10.34,19.15 10.64,18.85 10.64,13.06 v14.17,9.53
  Bottom 0.203: U2.28 11.99,23.92 11.99,23.57 12.98,22.58 12.98,20.32 11.81,19.15 v10.34,19.15
  Bottom 0.305: U3.5 16.64,7.06 v14.17,9.53
SPI_SCK  (via drill 0.3)
  Top 0.305: U1.SPI_CLK 7.16,21.72 7.59,21.29 v8.59,21.29
  $+3V3 0.305: v8.59,21.29 9.55,20.32 9.55,18.49 10.03,18.01 10.03,12.6 v13.23,9.4
  Bottom 0.203: v8.59,21.29 8.59,21.21 9.93,19.86 11.38,19.86 11.63,20.12 11.63,22.63 11.12,23.14 11.12,24.47 U2.26
  Bottom 0.305: U3.6 15.37,7.26 v13.23,9.4
TX  (via drill 0.3)
  $+3V3 0.305: v2.79,25.55 3.68,25.55 4.12,25.12 4.12,23.62 v7.34,20.4
  Bottom 0.203: v7.34,20.4 6.48,19.53 5.48,19.53 U2.12
  Bottom 0.305: JP1.3 1.68,26.67 v2.79,25.55
USB_DISC
  Bottom 0.203: U2.21 7.26,24.98 7.26,25.73 6.93,26.06 5.7,26.06 R7.2 R4.1
USBM  (via drill 0.3)
  Top 0.203: R6.1 12.94,28.73 16.18,28.73 16.71,28.19 16.71,24.92 v16.41,24.61
  Bottom 0.203: U2.32 14.5,23.6 15.39,23.6 v16.41,24.61
USBP  (via drill 0.3)
  Top 0.203: v17.09,23.44 17.04,23.39 8.61,23.39 7.75,24.26 7.75,25.88 7.42,26.21 7.42,28.54 R5.1
  Bottom 0.203: U2.33 14.8,23.19 16.84,23.19 v17.09,23.44
UVCC  (via drill 0.3)
  Top 0.406: 11.73,31.27 11.71,31.27 X1.VBUS
  Top 0.559: 11.73,31.27 12.6,31.27 13.08,31.75 v13.08,32.64
  Top 0.61: D1.2 v3.94,34.29
  $+3V3 0.813: v3.94,34.29 4.83,33.4 12.32,33.4 v13.08,32.64
  Bottom 0.61: v3.94,34.29 R1.2
VDDA  (via drill 0.3)
  $+3V3 0.305: v8.48,20.34 7.82,21.01 7.82,21.61 8.28,22.07 15.16,22.07 15.62,22.53 15.62,25.83 17.13,27.34
  $+3V3 0.813: JP2.3 17.8,26.67 17.13,27.34 16.74,27.74 16.74,31.77 v17.8,32.84
  Bottom 0.203: v8.48,20.34 8.42,20.34 U2.9 5.46,17.39 C14.1
  Bottom 0.813: L2.2 17.31,32.84 | 17.31,32.84 v17.8,32.84 | 17.31,32.84 17.31,34.13 C16.A
WIFI_CS  (via drill 0.3)
  Top 0.203: U1.SPI_CS 12.91,22.7
  Top 0.305: v10.97,20.52 11.33,20.17 12.6,20.17 13.03,20.6 13.03,22.33 U1.SPI_CS
  Bottom 0.203: U2.25 10.69,24.74 10.69,22.96 10.97,22.68 v10.97,20.52
WIFI_EN  (via drill 0.3)
  Top 0.203: 4.33,12.19 U1.VBAT_SW_EN
  Top 0.305: U1.VBAT_SW_EN 5.33,12.21 6.53,13.41 9.5,13.41 10.03,13.95 10.03,16.31 v9.17,17.17
  Bottom 0.203: U2.45 12.06,16.65 12.06,17.02 12.19,17.14 12.19,17.65 11.81,18.03 10.03,18.03 v9.17,17.17
WIFI_INT  (via drill 0.3)
  Top 0.305: v10.13,21.01 10.76,21.63 U1.SPI_IRQ
  Bottom 0.203: U2.22 10.13,22.82 v10.13,21.01

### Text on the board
tPlace: VCC | RAW | RST | GND | VDDA | TX | GND | BTN | RST | RX | D7 | A7 | D6 | A6 | D5 | A5 | D4 | A4 | D3 | A3 | D2 | A2 | D1 | A1 | D0 | A0

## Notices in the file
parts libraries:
SparkFun-Passives: Licensing: CC v3.0 Share-Alike You are welcome to use this library for commercial purposes.
